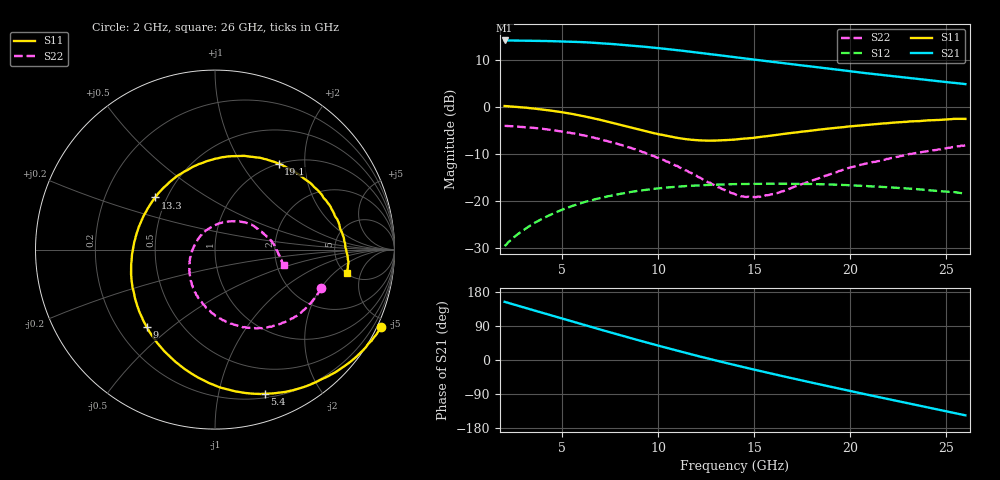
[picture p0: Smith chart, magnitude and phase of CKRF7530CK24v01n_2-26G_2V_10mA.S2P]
! CHUO DENSHI KOGYO Co.,Ltd.
! 14. January 2020
! CKRF7530CK24_RT5880
! N-channel HJ-FET
! Vds = 2 V, Id = 10 mA
# Hz S  MA  R 50
!	f	S11	S21	S12	S22
!	Hz	MAG	ANG	MAG	ANG	MAG	ANG	MAG	ANG
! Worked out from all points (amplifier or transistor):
!   241 points, 2 GHz to 26 GHz, reference 50 ohm
!   highest |S21| = 14.1 dB at 2 GHz (marker M1)
!   |S21| within 3 dB of that: start of sweep to 12.92 GHz
!   unconditionally stable (mu >= 1): 15.16 GHz to end of sweep
!   at 6 GHz: K = 0.51, MSG = 17.0 dB, |S12| = -20.3 dB
!   at 14 GHz: K = 0.97, MSG = 13.4 dB, |S12| = -16.4 dB
!   at 26 GHz: K = 1.13, MAG = 9.4 dB, |S12| = -18.4 dB
!   lowest NFmin = 0.59 dB at 18 GHz
!   S11 on the Smith chart (normalised r, x): 2 GHz: -0.23, -4.48; 5.4 GHz: 0.24, -1.37; 9 GHz: 0.32, -0.41; 13.3 GHz: 0.43, +0.31; 19.1 GHz: 1.00, +1.48; 26 GHz: 5.05, -2.99
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2e9  1.022 -25.1  5.055 153.6  0.03346 74.0  0.6301 -19.7
2.9e9  0.9887 -36.6  5.031 140.2  0.04822 65.0  0.6134 -28.0
3.8e9  0.9445 -48.5  4.999 127.0  0.0628 56.5  0.5906 -37.0
4.6e9  0.9022 -59.4  4.964 115.4  0.07525 48.8  0.5631 -45.1
5.4e9  0.8499 -71.0  4.908 103.7  0.0873 41.2  0.5333 -53.7
6e9  0.8056 -80.2  4.857 94.8  0.09607 35.2  0.5034 -60.2
6.7e9  0.7505 -91.2  4.773 84.5  0.105 28.5  0.4689 -68.1
7.3e9  0.7022 -100.9  4.684 75.8  0.1119 23.0  0.4369 -74.4
8.1e9  0.6396 -114.7  4.553 64.4  0.1207 15.5  0.3948 -84.0
9e9  0.5755 -131.3  4.391 51.7  0.1291 7.4  0.3437 -94.5
1e10  0.5139 -151.2  4.193 37.9  0.1368 -1.7  0.2888 -107.9
1.08e10  0.477 -168.1  4.029 27.1  0.1417 -8.7  0.2459 -120.0
1.16e10  0.4519 174.8  3.858 16.6  0.1457 -15.5  0.2035 -133.1
1.33e10  0.4419 138.9  3.5 -4.9  0.1506 -29.1  0.1355 -169.5
1.4e10  0.4512 125.6  3.361 -13.5  0.152 -34.5  0.119 171.3
1.6e10  0.5001 92.5  2.993 -37.1  0.1536 -49.4  0.1192 110.6
1.8e10  0.5613 66.3  2.674 -59.7  0.1524 -63.7  0.1656 68.8
1.91e10  0.596 53.5  2.513 -72.1  0.1503 -71.8  0.1978 52.6
2.04e10  0.6313 39.9  2.33 -86.3  0.1462 -81.0  0.2393 36.7
2.2e10  0.6735 24.6  2.136 -103.3  0.1406 -92.0  0.2809 19.0
2.39e10  0.7158 6.7  1.937 -123.8  0.1323 -105.4  0.3365 2.2
2.6e10  0.7461 -10.1  1.743 -146.0  0.1207 -119.8  0.392 -12.9
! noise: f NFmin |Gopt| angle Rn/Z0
1.8e+10  0.59  0.384  -96.8  0.1
1.85e+10  0.65  0.392  -89.7  0.11
1.9e+10  0.67  0.407  -80.5  0.13
2e+10  0.76  0.419  -68.8  0.17
2.05e+10  0.78  0.435  -60.4  0.19
2.1e+10  0.87  0.457  -54.5  0.22
2.2e+10  1.02  0.473  -41.8  0.27
2.25e+10  1.07  0.48  -35.6  0.3
2.3e+10  1.14  0.492  -27.8  0.34
2.4e+10  1.26  0.507  -16.2  0.39
